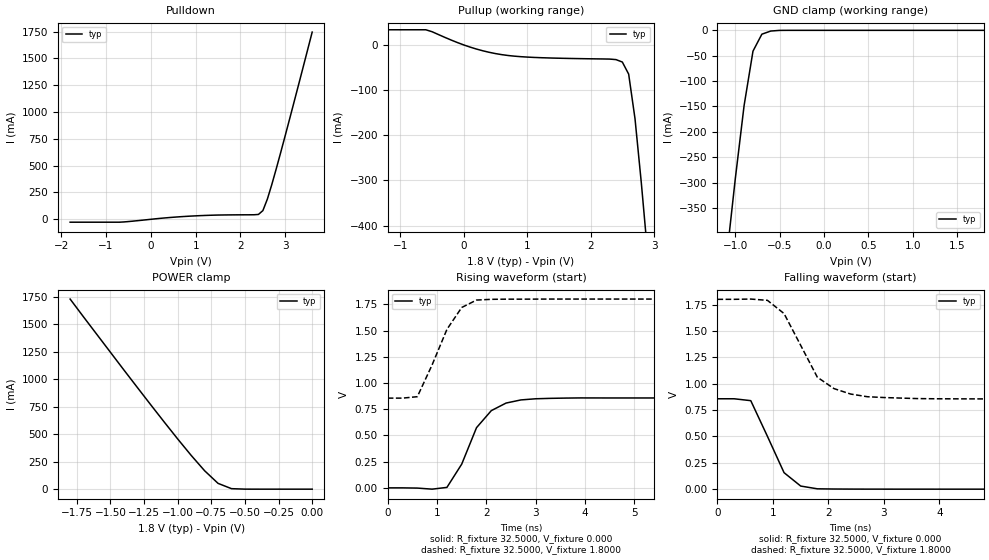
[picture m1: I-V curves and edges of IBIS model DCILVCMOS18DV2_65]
| / 7\'7
| \ \   Xilinx Inc.
| / /
| \_\/.\   IBIS Model for Virtex-II
[IBIS ver]   2.1
[File name]   dci1865d.ibs
[File Rev]   1.1
[Date]   Aug. 1, 2001
[Source]   Hspice simulations (08-1: TT, SS, FF)
[Notes]   Xilinx IBIS model for LVDCI 1.8V 32.5 ohms (65/2) driver
[Disclaimer] The data in this model is derived from SPICE simulations using
   modeling information extracted from the target process. While
   a great deal of care has been taken to provide information
   that is accurate, this model is considered preliminary as it
   has not been verified by actual silicon measurement. Treat the
   data in this model as preliminary until actual silicon
   verification is performed.
[Copyright]   Copyright 2001, Xilinx Inc., All rights reserved
|   Component Virtex_II
[Component]   Virtex_II
[Manufacturer]   Xilinx Inc.
[Package]
| variable   typ   min   max
R_pkg   0.1000   NA   NA
L_pkg   0.8000nH   NA   NA
C_pkg   0.5000pF   NA   NA
[Pin]  signal_name   model_name   R_pin   L_pin   C_pin
io   DCILVCMOS18DV2_65   DCILVCMOS18DV2_65
| ins  insig   inp
| ens  ensig   inp
PGND   GND   GND
VCCO   VCCO   POWER
| Models and submodels in the file (1): DCILVCMOS18DV2_65 (I/O)
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|   Model DCILVCMOS18DV2_65
[Model]   DCILVCMOS18DV2_65
Model_type   I/O
Polarity   Non-Inverting
Enable   Active-Low
Vinh = 1.19V
Vinl = 0.4V
Vmeas =   0.7900V
Cref =  35.0000pF
Rref =   1.0000M
Vref =  0.000V
C_comp   7.0000pF   NA   NA
[Temperature Range]   25.0000   NA   NA
[Voltage Range]   1.8000V   NA   NA
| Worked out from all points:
|   slope of the pulldown table from 0 to 0.27 V, typ, clamps not added: 24.2 ohm
|   slope of the pullup table from 0 to 0.27 V, typ, clamps not added: 22.9 ohm
|   GND clamp passes 1 mA (typ) near -0.57 V on its own axis
|   POWER clamp passes 1 mA (typ) near -0.52 V on its own axis
|   rising waveform, R_fixture 32.5000, V_fixture 0.000: 20-80 % time 581ps typ, NA min, NA max; typ from 0 V to 0.857 V
|   rising waveform, R_fixture 32.5000, V_fixture 1.8000: 20-80 % time 571ps typ, NA min, NA max; typ from 0.856 V to 1.8 V
|   falling waveform, R_fixture 32.5000, V_fixture 0.000: 20-80 % time 451ps typ, NA min, NA max; typ from 0.857 V to 0 V
|   falling waveform, R_fixture 32.5000, V_fixture 1.8000: 20-80 % time 594ps typ, NA min, NA max; typ from 1.8 V to 0.856 V
[Pulldown]
| voltage   I(typ)   I(min)   I(max)
-1.8V     -26.93mA   NA         NA
-700mV    -26.93mA   NA         NA
900mV     30.08mA    NA         NA
2.4V      45.18mA    NA         NA
2.5V      81.2mA     NA         NA
2.6V      188.3mA    NA         NA
2.7V      325.7mA    NA         NA
3V        783.4mA    NA         NA
3.6V      1.746A     NA         NA
[Pullup]
| voltage   I(typ)   I(min)   I(max)
-1.8V     33.63mA    NA         NA
-600mV    33.63mA    NA         NA
100mV     -4.789mA   NA         NA
600mV     -21.48mA   NA         NA
1.1V      -27.55mA   NA         NA
2.3V      -31.27mA   NA         NA
2.5V      -37.8mA    NA         NA
2.6V      -64.55mA   NA         NA
2.7V      -163.2mA   NA         NA
2.8V      -305.8mA   NA         NA
2.9V      -463.4mA   NA         NA
3.6V      -1.659A    NA         NA
[GND_clamp]
| voltage   I(typ)   I(min)   I(max)
-1.8V     -1.649A    NA         NA
-1.1V     -452.1mA   NA         NA
-1V       -293.4mA   NA         NA
-900mV    -148mA     NA         NA
-800mV    -41.01mA   NA         NA
-700mV    -7.602mA   NA         NA
-600mV    -1.419mA   NA         NA
-500mV    -128.9uA   NA         NA
1.8V      272.1nA    NA         NA
[POWER_clamp]
| voltage   I(typ)   I(min)   I(max)
-1.8V     1.731A     NA         NA
-1.4V     1.085A     NA         NA
-1V       456.9mA    NA         NA
-800mV    167.8mA    NA         NA
-700mV    52.78mA    NA         NA
-600mV    4.607mA    NA         NA
0V        272.1nA    NA         NA
[Ramp]
| variable   typ   min   max
dV/dt_r   0.5143/0.6086n   NA   NA
dV/dt_f   0.5666/0.6508n   NA   NA
R_load = 32.5000
[Rising Waveform]
R_fixture = 32.5000
V_fixture = 0.000
| time   V(typ)   V(min)   V(max)
0s        5.077uV    NA         NA
900ps     -12.41mV   NA         NA
1.2ns     4.533mV    NA         NA
1.5ns     226.3mV    NA         NA
1.8ns     573.8mV    NA         NA
2.1ns     736.4mV    NA         NA
2.4ns     808.6mV    NA         NA
2.7ns     838.4mV    NA         NA
3.9ns     857.5mV    NA         NA
15ns      857.1mV    NA         NA
[Rising Waveform]
R_fixture = 32.5000
V_fixture = 1.8000
V_fixture_min = 1.7000
V_fixture_max = 1.9000
| time   V(typ)   V(min)   V(max)
0s        855.6mV    NA         NA
300ps     855.6mV    NA         NA
600ps     869.2mV    NA         NA
900ps     1.173V     NA         NA
1.2ns     1.511V     NA         NA
1.5ns     1.72V      NA         NA
1.8ns     1.79V      NA         NA
2.1ns     1.798V     NA         NA
3.3ns     1.8V       NA         NA
15ns      1.8V       NA         NA
[Falling Waveform]
R_fixture = 32.5000
V_fixture = 0.000
| time   V(typ)   V(min)   V(max)
0s        857.1mV    NA         NA
300ps     857.1mV    NA         NA
600ps     839.2mV    NA         NA
900ps     501.4mV    NA         NA
1.2ns     156.4mV    NA         NA
1.5ns     29.45mV    NA         NA
1.8ns     3.333mV    NA         NA
3.6ns     49.76uV    NA         NA
15ns      -2.387uV   NA         NA
[Falling Waveform]
R_fixture = 32.5000
V_fixture = 1.8000
V_fixture_min = 1.7000
V_fixture_max = 1.9000
| time   V(typ)   V(min)   V(max)
0s        1.8V       NA         NA
600ps     1.802V     NA         NA
900ps     1.79V      NA         NA
1.2ns     1.665V     NA         NA
1.8ns     1.062V     NA         NA
2.1ns     953.6mV    NA         NA
2.4ns     902mV      NA         NA
2.7ns     876.6mV    NA         NA
4.2ns     856.6mV    NA         NA
15ns      855.6mV    NA         NA
